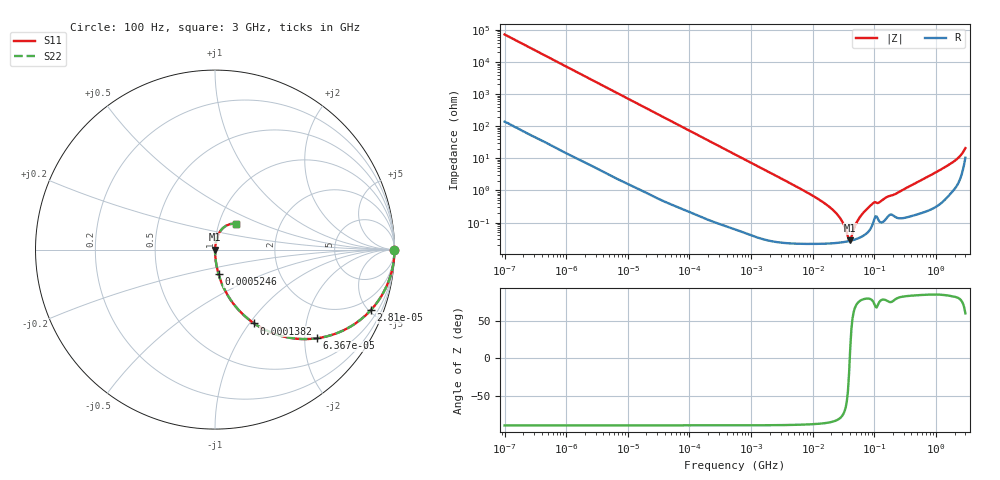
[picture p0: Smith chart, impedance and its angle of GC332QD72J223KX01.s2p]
!Murata Part Number: GC332QD72J223KX01
!These Parameters are Measured in Series Mode Connection
!Data Generated on Jan 08, 2026
!  o--ll--o
!Port1  Port2
!  o------o
!Operation Temp=25[degC], DC Bias Voltage=0[V]
!Freq. Start=100[Hz] Stop=3[GHz] 401[Steps]
# Hz S RI R 50
!Freq.(Hz) S11(Real) S11(Imag) S21(Real) S21(Imag) S12(Real) S12(Imag) S22(Real) S22(Imag)
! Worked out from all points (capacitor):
!   401 points, 100 Hz to 3 GHz, reference 50 ohm
!   read as one part in series: C = 22.1 nF near 109 Hz
!   lowest |Z| = 27.7 mohm at 40.54 MHz (marker M1)
!   series resonance near 39.91 MHz, so ESL is about 720 pH
!   S11 on the Smith chart (normalised r, x): 100 Hz: open; 28.1 kHz: 1.01, -5.17; 63.67 kHz: 1.01, -2.29; 138.2 kHz: 1.00, -1.05; 524.6 kHz: 1.00, -0.28; 3 GHz: 1.21, +0.36
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100  1 -0.00139  4.6e-06 0.00139  4.6e-06 0.00139  1 -0.00139
1788  0.9993 -0.0247  0.00066 0.0247  0.00066 0.0247  0.9993 -0.0247
8421  0.9865 -0.1145  0.0135 0.1145  0.0135 0.1145  0.9865 -0.1145
28103  0.8693 -0.3359  0.1307 0.3359  0.1307 0.3359  0.8693 -0.3359
31977  0.8373 -0.3679  0.1627 0.3679  0.1627 0.3679  0.8373 -0.3679
63668  0.5662 -0.4943  0.4338 0.4943  0.4338 0.4943  0.5662 -0.4943
138163  0.2183 -0.4115  0.7817 0.4115  0.7817 0.4115  0.2183 -0.4115
241767  0.0842 -0.2759  0.9158 0.2759  0.9158 0.2759  0.0842 -0.2759
524648  0.0196 -0.1364  0.9804 0.1364  0.9804 0.1364  0.0196 -0.1364
547723  0.0181 -0.1309  0.9819 0.1309  0.9819 0.1309  0.0181 -0.1309
9794414  0.000266 -0.00703  0.9997 0.00703  0.9997 0.00703  0.000266 -0.00703
2.418395e7  0.000236 -0.00192  0.9998 0.00192  0.9998 0.00192  0.000236 -0.00192
2.999103e7  0.000244 -0.00107  0.9998 0.00107  0.9998 0.00107  0.000244 -0.00107
3.71925e7  0.000261 -0.00026  0.9997 0.00026  0.9997 0.00026  0.000261 -0.00026
4.0536e7  0.000271 5.83e-05  0.9997 -5.83e-05  0.9997 -5.83e-05  0.000271 5.83e-05
5.248048e7  0.000316 0.00103  0.9997 -0.00103  0.9997 -0.00103  0.000316 0.00103
7.093284e7  0.00043 0.0023  0.9996 -0.0023  0.9996 -0.0023  0.00043 0.0023
9.587315e7  0.00102 0.00392  0.999 -0.00392  0.999 -0.00392  0.00102 0.00392
1.751444e8  0.00175 0.00651  0.9982 -0.00651  0.9982 -0.00651  0.00175 0.00651
1.506733e9  0.00923 0.0571  0.9908 -0.0571  0.9908 -0.0571  0.00923 0.0571
2.219584e9  0.0235 0.0927  0.9765 -0.0927  0.9765 -0.0927  0.0235 0.0927
3e9  0.1183 0.1446  0.8817 -0.1446  0.8817 -0.1446  0.1183 0.1446
